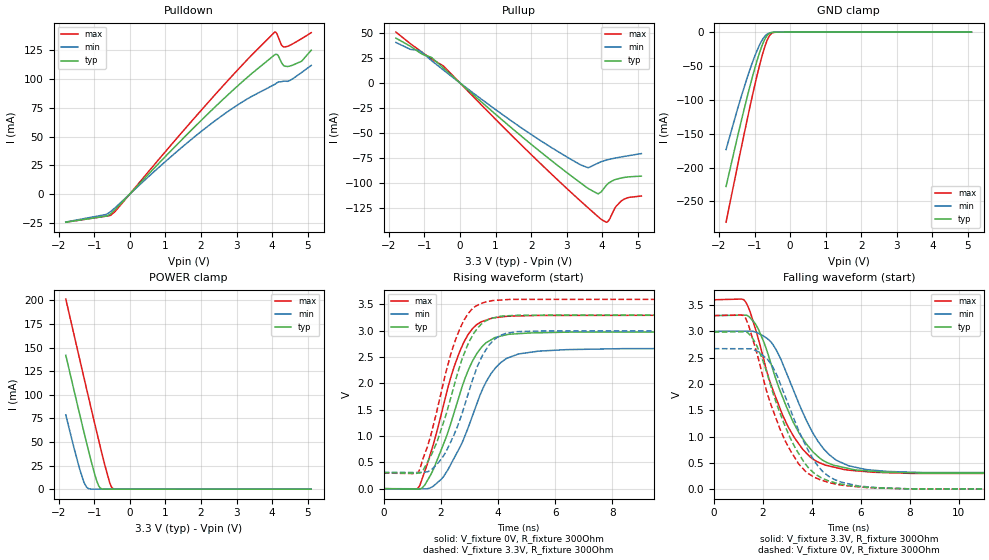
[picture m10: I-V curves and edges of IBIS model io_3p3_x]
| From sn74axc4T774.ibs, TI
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|   io_3p3_x Model
[Model]   io_3p3_x
Model_type   I/O
Polarity   Non-Inverting
Enable   Active-Low
Vinl = 0.8
Vinh = 2
Vmeas = 1.65
Vref = 0
Cref = 2pF
Rref = 100000
|   typ   min   max
C_comp   3.045pF   2.580pF   3.293pF
| Where Nom  PVT is Nominal Process, 3.3V, 27C
|   Fast PVT is Strong Process,  3.6V, -40C
|   Slow PVT is Weak Process,   3.0V, 130C
[Voltage Range]   3.3   3   3.6
|Junction Temperature
[Temperature Range]   27   130   -40
[Pullup Reference]   3.3   3   3.6
[Pulldown Reference]   0   -0   -0
[Power Clamp Reference]   3.3   3   3.6
[GND Clamp Reference]   0   0   0
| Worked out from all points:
|   slope of the pulldown table from 0 to 0.495 V, typ, clamps not added: 30.3 ohm
|   slope of the pullup table from 0 to 0.495 V, typ, clamps not added: 31.8 ohm
|   GND clamp passes 1 mA (typ) near -0.54 V on its own axis
|   POWER clamp passes 1 mA (typ) near -0.83 V on its own axis
|   falling waveform, V_fixture 3.3V, R_fixture 300Ohm: 20-80 % time 1.6ns typ, 1.61ns min, 1.55ns max; typ from 3.3 V to 0.302 V
|   rising waveform, V_fixture 0V, R_fixture 300Ohm: 20-80 % time 1.17ns typ, 1.28ns min, 1.05ns max; typ from 0 V to 2.98 V
|   rising waveform, V_fixture 3.3V, R_fixture 300Ohm: 20-80 % time 1.04ns typ, 1.08ns min, 973ps max; typ from 0.302 V to 3.3 V
|   falling waveform, V_fixture 0V, R_fixture 300Ohm: 20-80 % time 1.53ns typ, 1.51ns min, 1.5ns max; typ from 2.98 V to 0 V
[Pulldown]
|   Voltage   I(typ)   I(min)   I(max)
-1.8V     -24.53mA   -24.37mA   -24.52mA
-675.3mV  -19.29mA   -17.85mA   -19.3mA
-420mV    -13.8mA    -12.15mA   -15.42mA
2.14V     68.14mA    57.7mA     77.54mA
3.106V    96.16mA    79.01mA    110.5mA
4.072V    121.1mA    95.41mA    140.9mA
4.168V    120.6mA    97.37mA    137mA
4.265V    114.4mA    97.81mA    129.6mA
4.348V    111.4mA    98.36mA    128mA
4.507V    111.4mA    98.96mA    129.5mA
4.831V    115.6mA    105.8mA    135.2mA
5.1V      125.2mA    111.9mA    140.4mA
[GND Clamp]
|   Voltage   I(typ)   I(min)   I(max)
-1.8V     -227.8mA   -173.4mA   -280.6mA
-1.372V   -131.2mA   -95.11mA   -170.7mA
-1.151V   -84.56mA   -58.82mA   -115.9mA
-944.4mV  -44.95mA   -29.29mA   -67.54mA
-813.3mV  -23.61mA   -14.42mA   -40.11mA
-709.8mV  -10.58mA   -6.214mA   -21.59mA
-606.3mV  -2.952mA   -1.889mA   -7.765mA
-516.6mV  -668.4uA   -524.4uA   -1.826mA
-406.2mV  -131.4uA   -108.9uA   -233.1uA
-68.1mV   -1.279uA   -1.561uA   -1.232uA
5.1V      0A         0A         0A
[Pullup]
|   Voltage   I(typ)   I(min)   I(max)
-1.8V     44.59mA    40.29mA    50.61mA
-1.131V   30.15mA    32.18mA    32.25mA
-468.3mV  14.94mA    12.9mA     16.97mA
1.56V     -48.11mA   -40.68mA   -56.01mA
3.209V    -94.78mA   -77.95mA   -111.8mA
3.61V     -105.3mA   -84.49mA   -124.7mA
3.879V    -110.5mA   -79.95mA   -133.1mA
3.975V    -108.3mA   -78.39mA   -136mA
4.162V    -100.4mA   -76.4mA    -138mA
4.389V    -96mA      -74.69mA   -122.9mA
4.638V    -94.05mA   -73.12mA   -115.4mA
5.1V      -92.82mA   -70.4mA    -112.7mA
[POWER Clamp]
|   Voltage   I(typ)   I(min)   I(max)
-1.8V     141.9mA    78.74mA    201.4mA
-1.565V   104.1mA    43.12mA    163mA
-1.407V   78.83mA    20.87mA    137.2mA
-1.296V   61.5mA     8.016mA    119.2mA
-1.214V   48.71mA    2.066mA    105.8mA
-985.8mV  15.65mA    4.518uA    69.3mA
-868.5mV  3.093mA    456.3nA    50.79mA
-771.9mV  146.4uA    317.2nA    35.85mA
-571.8mV  159.9nA    299.2nA    7.669mA
-516.6mV  99.77nA    296.5nA    2.383mA
-468.3mV  91.36nA    293.9nA    390.4uA
5.1V      0A         0A         0A
[Ramp]
R_load = 300
|   typ   min   max
dV/dt_r   1.79089/1.16187e-09   1.60246/1.27794e-09   1.97921/1.04954e-09
dV/dt_f   1.79877/1.59447e-09   1.61386/1.59958e-09   1.98258/1.55125e-09
[Falling Waveform]
V_fixture = 3.3V
V_fixture_min = 3V
V_fixture_max = 3.6V
R_fixture = 300Ohm
C_fixture = 0F
|   Time   V(typ)   V(min)   V(max)
0s        3.3V       3V         3.6V
1.303ns   3.308V     3.003V     3.558V
1.828ns   3.033V     2.96V      2.839V
2.388ns   2.306V     2.765V     1.918V
3.031ns   1.494V     2.133V     1.185V
3.919ns   779.5mV    1.177V     617.4mV
4.705ns   489.1mV    657.6mV    440.4mV
5.507ns   391.9mV    444.1mV    361mV
8.067ns   311.1mV    322.8mV    299.6mV
500ns     302mV      310.2mV    295.7mV
[Rising Waveform]
V_fixture = 0V
V_fixture_min = 0V
V_fixture_max = 0V
R_fixture = 300Ohm
C_fixture = 0F
|   Time   V(typ)   V(min)   V(max)
0s        177.7nV    701.8nV    89.21nV
1.251ns   -8.06mV    -2.837mV   47.08mV
1.647ns   264.6mV    20.6mV     681.3mV
2.088ns   841.3mV    225.4mV    1.574V
2.641ns   1.757V     761mV      2.58V
3.105ns   2.421V     1.383V     3.038V
3.478ns   2.718V     1.912V     3.18V
3.93ns    2.875V     2.306V     3.249V
5.312ns   2.959V     2.603V     3.288V
500ns     2.985V     2.671V     3.299V
[Rising Waveform]
V_fixture = 3.3V
V_fixture_min = 3V
V_fixture_max = 3.6V
R_fixture = 300Ohm
C_fixture = 0F
|   Time   V(typ)   V(min)   V(max)
0s        302mV      310.2mV    295.7mV
1.217ns   295.5mV    306.7mV    319.3mV
1.374ns   343.1mV    306.2mV    569.4mV
1.931ns   992.5mV    504.1mV    1.638V
2.456ns   1.94V      1.017V     2.738V
2.932ns   2.723V     1.76V      3.307V
3.29ns    3.052V     2.338V     3.486V
3.676ns   3.214V     2.72V      3.557V
4.45ns    3.286V     2.964V     3.595V
500ns     3.3V       3V         3.6V
[Falling Waveform]
|Gnd
V_fixture = 0V
V_fixture_min = 0V
V_fixture_max = 0V
R_fixture = 300Ohm
C_fixture = 0F
|   Time   V(typ)   V(min)   V(max)
0s        2.985V     2.671V     3.299V
1.286ns   2.991V     2.669V     3.26V
1.763ns   2.718V     2.623V     2.578V
2.388ns   1.87V      2.34V      1.537V
2.909ns   1.201V     1.769V     920.6mV
3.745ns   474.3mV    833.2mV    336.3mV
4.258ns   252.3mV    433.1mV    194.8mV
4.913ns   125.7mV    185.8mV    104.1mV
8.067ns   4.801mV    5.947mV    3.376mV
500ns     187.5nV    726.1nV    97.74nV
